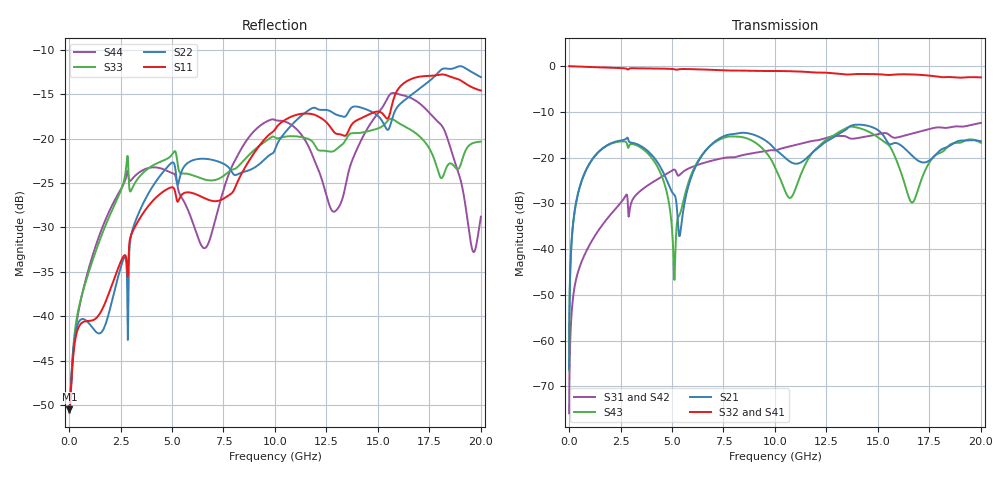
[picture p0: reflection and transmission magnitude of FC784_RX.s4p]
! Touchstone generated by fitter/viewer
# HZ S  RI R 5.000000e+001
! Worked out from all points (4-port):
!   4999 points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, 4.001 MHz to 20 GHz, reference 50 ohm
!   strongest paths, dB at 4.001 MHz, 5.001 GHz, 10 GHz, 15 GHz, 20 GHz:
!     S32: 0.0, -0.6, -1.1, -1.8, -2.5
!     S41: 0.0, -0.6, -1.1, -1.8, -2.4
!     S21: -66.1, -27.5, -18.2, -14.0, -16.4
!     S43: -66.6, -35.6, -22.2, -15.6, -16.8
!     S31: -75.9, -22.8, -18.4, -14.9, -12.4
!     S42: -76.5, -22.7, -18.5, -14.9, -12.5
!   lowest |S11| = -50.5 dB at 20 MHz (marker M1), VSWR 1.01, Z = 50.3 + j0.0263 ohm
!   |S11| at or under -10 dB: start of sweep to end of sweep
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4000800  0.00311 5.62e-06  0.000157 0.000468  -0.000132 -9.21e-05  0.9966 -0.00269
         0.000157 0.000468  0.00312 5.31e-05  0.9966 -0.00272  -0.00013 -7.4e-05
         -0.000132 -9.21e-05  0.9966 -0.00272  0.00309 -1.32e-05  0.000143 0.000443
         0.9966 -0.00269  -0.00013 -7.4e-05  0.000143 0.000443  0.00308 -4.17e-05
2.0004e7  0.00297 0.000261  0.00036 0.00209  -0.000205 -0.000372  0.996 -0.0127
          0.00036 0.00209  0.00306 0.00039  0.9959 -0.0128  -0.000157 -0.000346
          -0.000205 -0.000372  0.9959 -0.0128  0.00288 0.000276  0.000293 0.00204
          0.996 -0.0127  -0.000157 -0.000346  0.000293 0.00204  0.00284 0.000171
1.560312e9  -0.00548 -0.00913  0.0928 0.0802  -0.0135 -0.0113  0.6061 -0.7532
            0.0928 0.0802  -0.00171 -0.00791  0.6007 -0.7575  -0.0131 -0.0113
            -0.0135 -0.0113  0.6007 -0.7575  0.0136 -0.0246  0.0986 0.0715
            0.6061 -0.7532  -0.0131 -0.0113  0.0986 0.0715  0.0119 -0.0279
5.485097e9  0.0327 0.0357  0.0132 0.0164  -0.00229 0.0685  -0.9287 -0.0624
            0.0132 0.0164  0.0288 0.0595  -0.9263 -0.0471  -3.96e-05 0.0691
            -0.00229 0.0685  -0.9263 -0.0471  -0.0346 0.0533  0.0168 0.0235
            -0.9287 -0.0624  -3.96e-05 0.0691  0.0168 0.0235  -0.0406 0.0221
1.093019e10  0.1347 0.00226  0.0861 0.00407  0.00484 -0.1361  0.8628 0.1491
             0.0861 0.00407  0.1147 0.0453  0.8685 0.1086  0.00879 -0.1385
             0.00484 -0.1361  0.8685 0.1086  -0.0982 0.0311  -0.0357 0.0217
             0.8628 0.1491  0.00879 -0.1385  -0.0357 0.0217  -0.1121 -0.0311
1.645129e10  0.1895 -0.0946  0.0978 -0.0636  -0.0014 0.1777  -0.7819 -0.2043
             0.0978 -0.0636  0.165 -0.0405  -0.7997 -0.1414  -0.00246 0.1808
             -0.0014 0.1777  -0.7997 -0.1414  -0.1079 -0.0381  -0.0331 -0.0219
             -0.7819 -0.2043  -0.00246 0.1808  -0.0331 -0.0219  -0.1127 -0.1299
2e10  0.0963 -0.1597  0.1315 -0.0736  0.2141 -0.1063  0.1415 0.748
      0.1315 -0.0736  0.1174 -0.1879  0.1975 0.7262  0.2159 -0.101
      0.2141 -0.1063  0.1975 0.7262  0.0936 0.0219  0.1393 -0.0396
      0.1415 0.748  0.2159 -0.101  0.1393 -0.0396  0.0359 -0.00514
